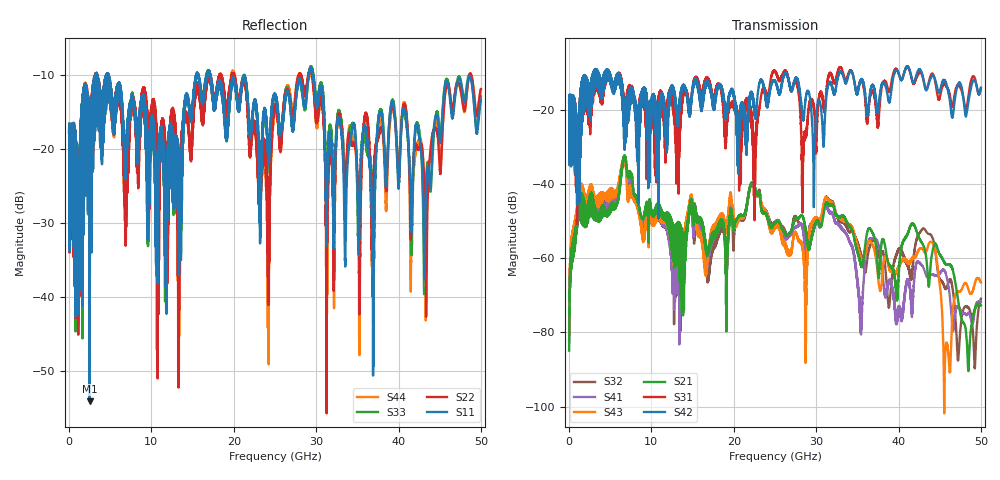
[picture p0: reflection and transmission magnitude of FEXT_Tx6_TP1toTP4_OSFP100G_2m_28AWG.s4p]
! Touchstone data
! Created: 27-Feb-2019 by IdEM 12 (12.1.0)
! COMMENTS
!  Created Wed Feb 27 12:03:36 2019
!  64 Port Network Data from SP1.SP block
!  freq  magS1_1  angS1_1  magS1_2  angS1_2  magS1_3  angS1_3  magS1_4  angS1_4
!  magS1_5  angS1_5  magS1_6  angS1_6  magS1_7  angS1_7  magS1_8  angS1_8
!  magS1_9  angS1_9  magS1_10  angS1_10  magS1_11  angS1_11  magS1_12  angS1_12
!  magS1_13  angS1_13  magS1_14  angS1_14  magS1_15  angS1_15  magS1_16  angS1_16
!  magS1_17  angS1_17  magS1_18  angS1_18  magS1_19  angS1_19  magS1_20  angS1_20
!  magS1_21  angS1_21  magS1_22  angS1_22  magS1_23  angS1_23  magS1_24  angS1_24
!  magS1_25  angS1_25  magS1_26  angS1_26  magS1_27  angS1_27  magS1_28  angS1_28
!  magS1_29  angS1_29  magS1_30  angS1_30  magS1_31  angS1_31  magS1_32  angS1_32
!  magS1_33  angS1_33  magS1_34  angS1_34  magS1_35  angS1_35  magS1_36  angS1_36
!  magS1_37  angS1_37  magS1_38  angS1_38  magS1_39  angS1_39  magS1_40  angS1_40
!  magS1_41  angS1_41  magS1_42  angS1_42  magS1_43  angS1_43  magS1_44  angS1_44
!  magS1_45  angS1_45  magS1_46  angS1_46  magS1_47  angS1_47  magS1_48  angS1_48
!  magS1_49  angS1_49  magS1_50  angS1_50  magS1_51  angS1_51  magS1_52  angS1_52
!  magS1_53  angS1_53  magS1_54  angS1_54  magS1_55  angS1_55  magS1_56  angS1_56
!  magS1_57  angS1_57  magS1_58  angS1_58  magS1_59  angS1_59  magS1_60  angS1_60
!  magS1_61  angS1_61  magS1_62  angS1_62  magS1_63  angS1_63  magS1_64  angS1_64
!  magS2_1  angS2_1  magS2_2  angS2_2  magS2_3  angS2_3  magS2_4  angS2_4
!  magS2_5  angS2_5  magS2_6  angS2_6  magS2_7  angS2_7  magS2_8  angS2_8
!  magS2_9  angS2_9  magS2_10  angS2_10  magS2_11  angS2_11  magS2_12  angS2_12
!  magS2_13  angS2_13  magS2_14  angS2_14  magS2_15  angS2_15  magS2_16  angS2_16
!  magS2_17  angS2_17  magS2_18  angS2_18  magS2_19  angS2_19  magS2_20  angS2_20
!  magS2_21  angS2_21  magS2_22  angS2_22  magS2_23  angS2_23  magS2_24  angS2_24
!  magS2_25  angS2_25  magS2_26  angS2_26  magS2_27  angS2_27  magS2_28  angS2_28
!  magS2_29  angS2_29  magS2_30  angS2_30  magS2_31  angS2_31  magS2_32  angS2_32
!  magS2_33  angS2_33  magS2_34  angS2_34  magS2_35  angS2_35  magS2_36  angS2_36
!  magS2_37  angS2_37  magS2_38  angS2_38  magS2_39  angS2_39  magS2_40  angS2_40
!  magS2_41  angS2_41  magS2_42  angS2_42  magS2_43  angS2_43  magS2_44  angS2_44
!  magS2_45  angS2_45  magS2_46  angS2_46  magS2_47  angS2_47  magS2_48  angS2_48
!  magS2_49  angS2_49  magS2_50  angS2_50  magS2_51  angS2_51  magS2_52  angS2_52
!  magS2_53  angS2_53  magS2_54  angS2_54  magS2_55  angS2_55  magS2_56  angS2_56
!  magS2_57  angS2_57  magS2_58  angS2_58  magS2_59  angS2_59  magS2_60  angS2_60
!  magS2_61  angS2_61  magS2_62  angS2_62  magS2_63  angS2_63  magS2_64  angS2_64
!  magS3_1  angS3_1  magS3_2  angS3_2  magS3_3  angS3_3  magS3_4  angS3_4
!  magS3_5  angS3_5  magS3_6  angS3_6  magS3_7  angS3_7  magS3_8  angS3_8
!  magS3_9  angS3_9  magS3_10  angS3_10  magS3_11  angS3_11  magS3_12  angS3_12
!  magS3_13  angS3_13  magS3_14  angS3_14  magS3_15  angS3_15  magS3_16  angS3_16
!  magS3_17  angS3_17  magS3_18  angS3_18  magS3_19  angS3_19  magS3_20  angS3_20
!  magS3_21  angS3_21  magS3_22  angS3_22  magS3_23  angS3_23  magS3_24  angS3_24
!  magS3_25  angS3_25  magS3_26  angS3_26  magS3_27  angS3_27  magS3_28  angS3_28
!  magS3_29  angS3_29  magS3_30  angS3_30  magS3_31  angS3_31  magS3_32  angS3_32
!  magS3_33  angS3_33  magS3_34  angS3_34  magS3_35  angS3_35  magS3_36  angS3_36
!  magS3_37  angS3_37  magS3_38  angS3_38  magS3_39  angS3_39  magS3_40  angS3_40
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# Hz S MA R 50
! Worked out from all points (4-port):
!   5000 points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, 10 MHz to 50 GHz, reference 50 ohm
!   strongest paths, dB at 10 MHz, 12.51 GHz, 25.01 GHz, 37.51 GHz, 50 GHz:
!     S42: -18.0, -14.6, -12.2, -20.3, -14.0
!     S31: -18.0, -16.4, -9.6, -24.1, -14.3
!     S21: -84.9, -50.5, -50.5, -63.8, -72.7
!     S43: -80.6, -52.1, -51.4, -65.0, -66.6
!     S41: -82.7, -53.2, -50.3, -55.8, -71.8
!     S32: -82.5, -52.9, -50.3, -58.2, -71.0
!   lowest |S11| = -54.1 dB at 2.49 GHz (marker M1), VSWR 1.00, Z = 49.8 + j0.0446 ohm
!   |S11| at or under -10 dB: 4.81 GHz to 15.41 GHz (10.6 GHz wide, 105 % of centre); 17.19 GHz to 29.09 GHz (11.9 GHz wide, 51.4 % of centre); 29.64 GHz to end of sweep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
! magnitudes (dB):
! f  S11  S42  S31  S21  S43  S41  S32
! 10 MHz  -17.7  -18.0  -18.0  -84.9  -80.6  -82.7  -82.5
! 2.49 GHz  -54.1  -20.1  -22.3  -48.4  -45.8  -47.1  -46.8
! 31.31 GHz  -25.2  -15.1  -13.8  -45.3  -44.0  -46.5  -43.7
! 38.84 GHz  -17.1  -17.9  -15.2  -61.6  -62.3  -66.0  -73.2
! 43.37 GHz  -24.7  -14.8  -14.6  -60.0  -58.3  -64.8  -52.9
! 45.65 GHz  -11.4  -12.3  -13.2  -61.4  -86.9  -63.6  -68.1
! 50 GHz  -13.3  -14.0  -14.3  -72.7  -66.6  -71.8  -71.0
